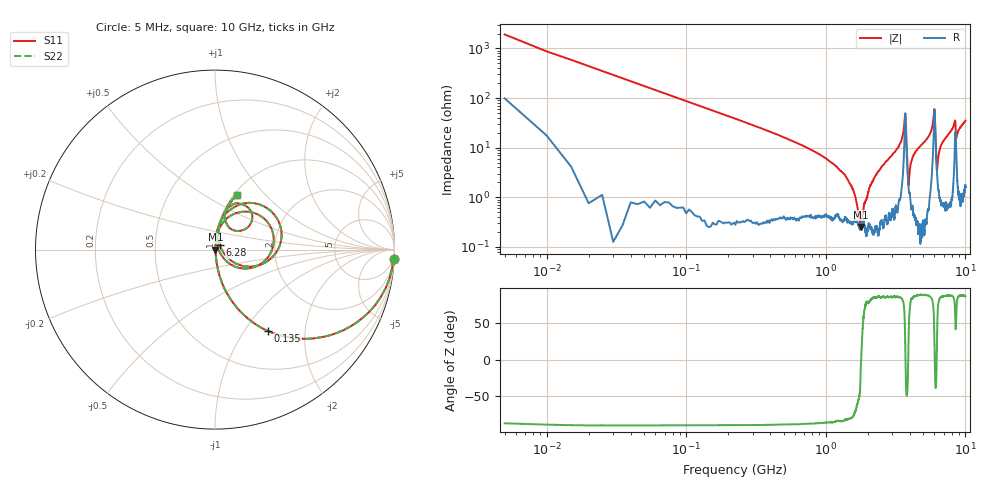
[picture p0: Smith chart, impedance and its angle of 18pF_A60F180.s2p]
! Amotech Co.,Ltd.
! http://www.amotech.co.kr/
! Part Number: A60F180
! These Parameters are Measured in Series Mode Connection
! Operation Temp=25[degC], DC Bias Voltage=0[V]
! Freq. Start=5[MHz] Stop=10[GHz], 2000[Steps]
! Date: Monday, July 20, 2020, 03:36:01
# GHZ S RI R 50.000000
!Freq.(Hz) S11(Real) S11(Imag) S21(Real) S21(Imag) S12(Real) S12(Imag) S22(Real) S22(Imag)
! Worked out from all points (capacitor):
!   2000 points, 5 MHz to 10 GHz, reference 50 ohm
!   read as one part in series: C = 18.2 pF near 55 MHz
!   lowest |Z| = 254 mohm at 1.795 GHz (marker M1)
!   series resonance near 1.793 GHz, so ESL is about 430 pH
!   S11 on the Smith chart (normalised r, x): 5 MHz: 3, -38; 135 MHz: 1.01, -1.29; 6.28 GHz: 1.05, +0.05; 10 GHz: 1.04, +0.70
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0.005  0.9946 -0.0518  0.0054 0.0518  0.0054 0.0518  0.9946 -0.0518
0.07  0.6081 -0.485  0.3919 0.485  0.3919 0.485  0.6081 -0.485
0.135  0.295 -0.4534  0.705 0.4534  0.705 0.4534  0.295 -0.4534
0.38  0.0496 -0.2095  0.9504 0.2095  0.9504 0.2095  0.0496 -0.2095
1.375  0.0043 -0.0272  0.9957 0.0272  0.9957 0.0272  0.0043 -0.0272
1.675  0.00331 -0.00602  0.9967 0.00602  0.9967 0.00602  0.00331 -0.00602
1.795  0.00253 0.000151  0.9975 -0.000151  0.9975 -0.000151  0.00253 0.000151
2.24  0.00262 0.0254  0.9974 -0.0254  0.9974 -0.0254  0.00262 0.0254
3.34  0.0199 0.1041  0.9801 -0.1041  0.9801 -0.1041  0.0199 0.1041
3.705  0.3256 0.0796  0.6744 -0.0796  0.6744 -0.0796  0.3256 0.0796
3.92  0.0149 0.00963  0.9851 -0.00963  0.9851 -0.00963  0.0149 0.00963
4.225  0.00953 0.0682  0.9905 -0.0682  0.9905 -0.0682  0.00953 0.0682
5.005  0.0186 0.1232  0.9814 -0.1232  0.9814 -0.1232  0.0186 0.1232
5.735  0.0728 0.2125  0.9272 -0.2125  0.9272 -0.2125  0.0728 0.2125
5.985  0.3598 0.1437  0.6402 -0.1437  0.6402 -0.1437  0.3598 0.1437
6.085  0.1848 -0.095  0.8152 0.095  0.8152 0.095  0.1848 -0.095
6.215  0.0416 -0.0079  0.9584 0.0079  0.9584 0.0079  0.0416 -0.0079
6.28  0.0271 0.0236  0.9729 -0.0236  0.9729 -0.0236  0.0271 0.0236
6.67  0.0195 0.1055  0.9805 -0.1055  0.9805 -0.1055  0.0195 0.1055
8.335  0.1244 0.2586  0.8756 -0.2586  0.8756 -0.2586  0.1244 0.2586
8.605  0.0794 0.1218  0.9206 -0.1218  0.9206 -0.1218  0.0794 0.1218
10  0.1213 0.302  0.8787 -0.302  0.8787 -0.302  0.1213 0.302
